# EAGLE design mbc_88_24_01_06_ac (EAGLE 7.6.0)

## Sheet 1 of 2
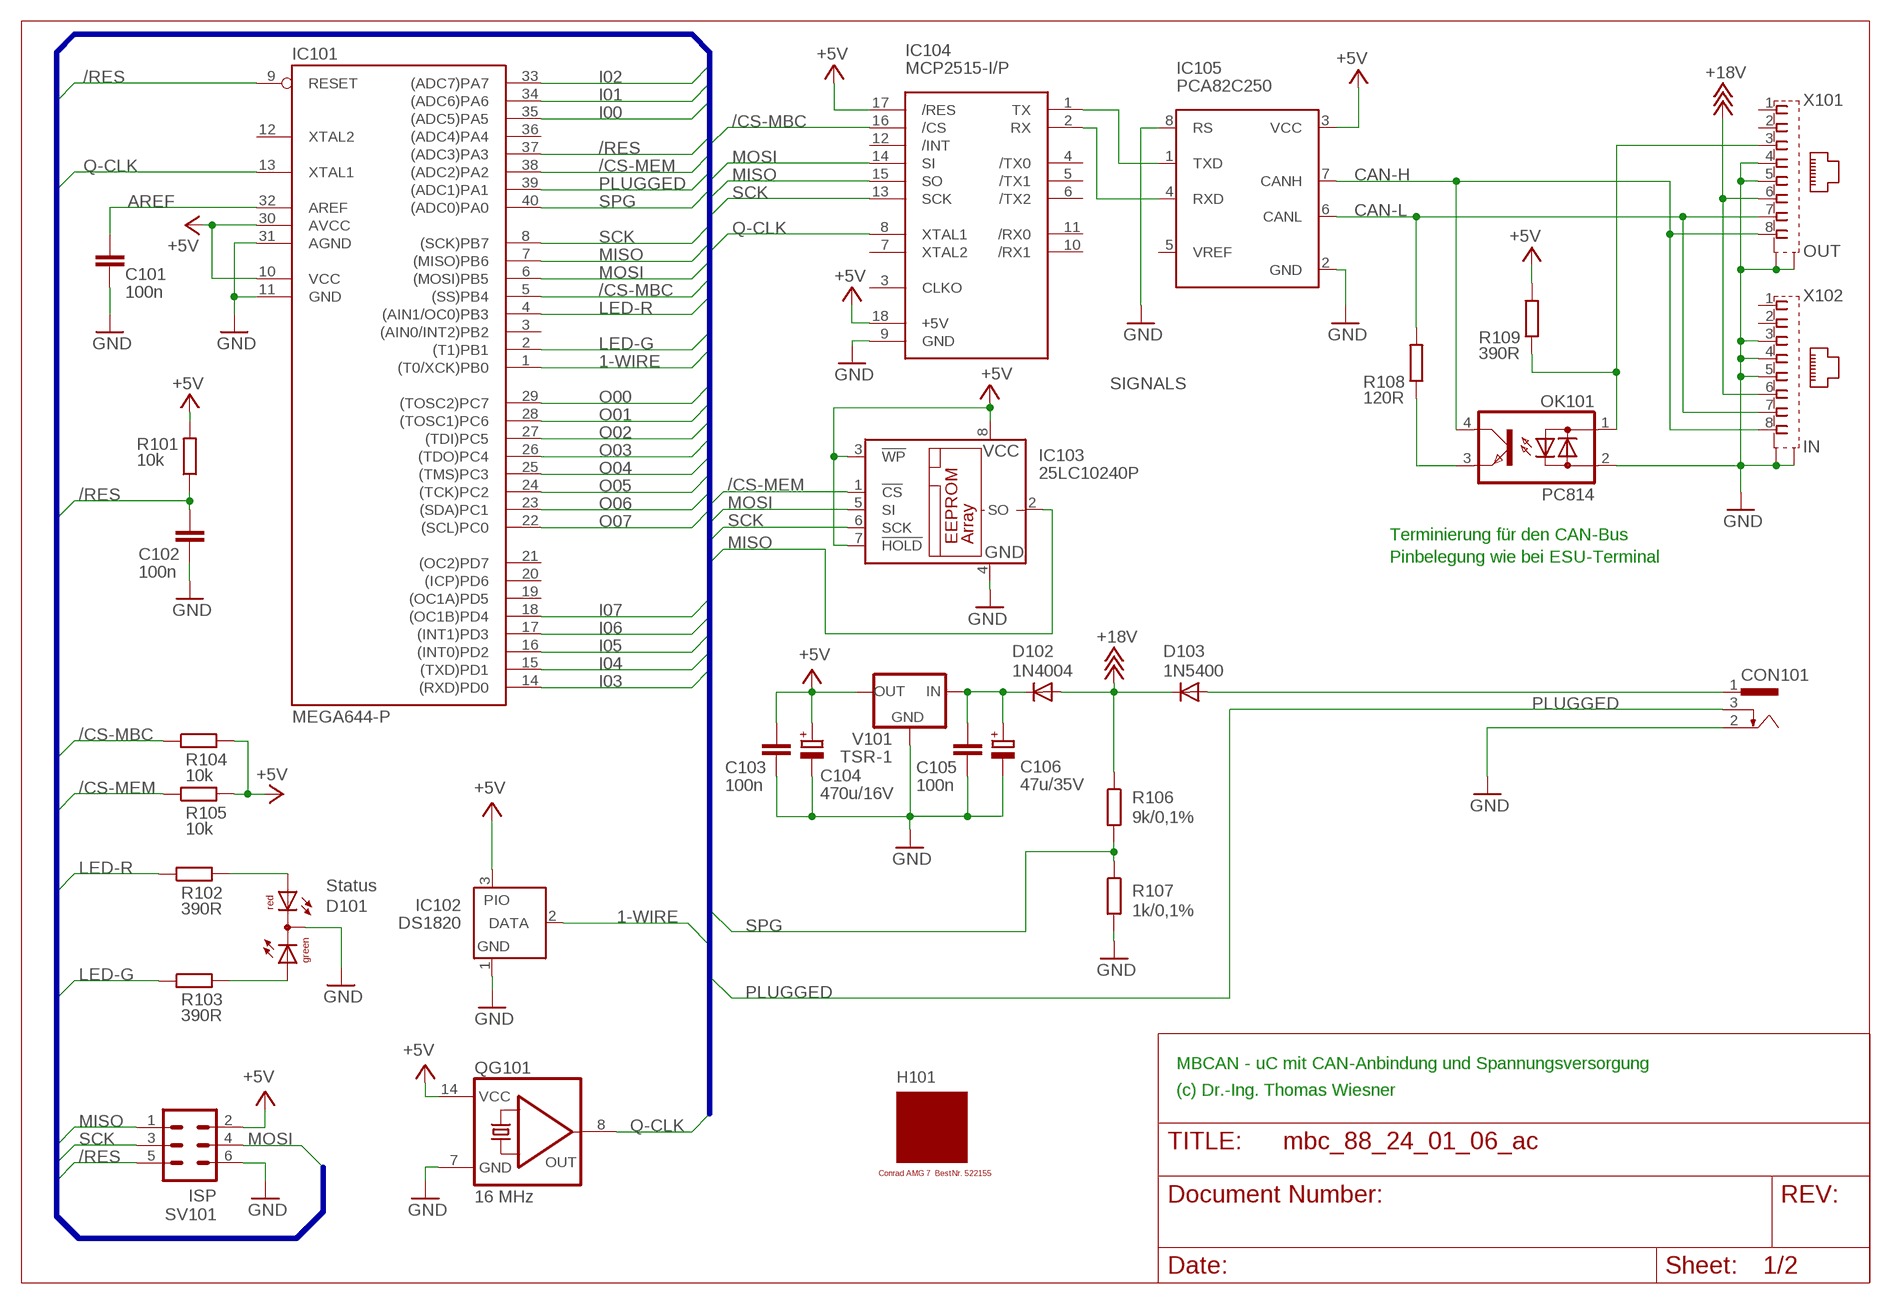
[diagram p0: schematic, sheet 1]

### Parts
C101  100n  C-EU025-025X050  [C025-025X050]
C102  100n  C-EU025-025X050  [C025-025X050]
C103  100n  C-EU025-025X050  [C025-025X050]
C104  470u/16V  CPOL-EUE3.5-8  [E3,5-8]
C105  100n  C-EU025-025X050  [C025-025X050]
C106  47u/35V  CPOL-EUE2.5-7  [E2,5-7]
CON101  POWER-JACK  [POWER-JACK]
D101  Status  DUOLED5MM  [DUOLED5MM]
D102  1N4004  [DO41-10]
D103  1N5400  [DO201-15]
H101  MODULGEHÄUSE-AMG-7  [MODULGEHÄUSE-1]
IC101  MEGA644-P  MEGA323-P  [DIL40]
IC102  DS1820  DS2405  [TO92-]
IC103  25LC10240P  25LC040P  [DIL8]
IC104  MCP2515-I/P  MCP2510-I/P  [DIL18]
IC105  PCA82C250  [DIL08]
OK101  PC814  [DIL04]
QG101  16 MHz  QG5860  [DIL14S]
R101  10k  R-EU_0207/10  [0207/10]
R102  390R  R-EU_0207/10  [0207/10]
R103  390R  R-EU_0207/10  [0207/10]
R104  10k  R-EU_0207/10  [0207/10]
R105  10k  R-EU_0207/10  [0207/10]
R106  9k/0,1%  R-EU_0207/10  [0207/10]
R107  1k/0,1%  R-EU_0207/10  [0207/10]
R108  120R  R-EU_0207/10  [0207/10]
R109  390R  R-EU_0207/10  [0207/10]
SV101  ISP  ML6  [ML6]
V101  TSR-1  [TRACO-TSR-1]
X101  OUT  0446200002  [0446200002]
X102  IN  0446200002  [0446200002]

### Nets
1-WIRE: IC101.1((T0/XCK)PB0) IC102.2(DATA)
+5V: C103.1 C104.+ IC101.10(VCC) IC101.30(AVCC) IC102.3(PIO) IC103.3(!WP) IC103.7(!HOLD) IC103.8(VCC) IC104.17(/RES) IC104.18(+5V) IC105.3(VCC) QG101.14(VCC) R101.2 R104.2 R105.2 R109.2 SV101.2 V101.OUT ; also sheet 2
+18V: D102.A D103.C R106.1 X101.6 X102.6
/CS-MBC: IC101.5((SS)PB4) IC104.16(/CS) R104.1
/CS-MEM: IC101.38((ADC2)PA2) IC103.1(!CS) R105.1
/RES: C102.1 IC101.9(RESET) IC101.37((ADC3)PA3) R101.1 SV101.5
AREF: C101.1 IC101.32(AREF)
CAN-H: IC105.7(CANH) OK101.4(C) X101.8 X102.8
CAN-L: IC105.6(CANL) R108.2 X101.7 X102.7
GND: C101.2 C102.2 C103.2 C104.- C105.2 C106.- CON101.2 D101.K(C) IC101.11(GND) IC101.31(AGND) IC102.1(GND) IC103.4(GND) IC104.9(GND) IC105.2(GND) IC105.8(RS) OK101.2(AC2) QG101.7(GND) R107.2 SV101.6 V101.GND X101.4 X101.5 X101.S@1(S1) X101.S@2(S2) X102.3 X102.4 X102.5 X102.S@1(S1) X102.S@2(S2) ; also sheet 2
I00: IC101.35((ADC5)PA5) ; also sheet 2
I01: IC101.34((ADC6)PA6) ; also sheet 2
I02: IC101.33((ADC7)PA7) ; also sheet 2
I03: IC101.14((RXD)PD0) ; also sheet 2
I04: IC101.15((TXD)PD1) ; also sheet 2
I05: IC101.16((INT0)PD2) ; also sheet 2
I06: IC101.17((INT1)PD3) ; also sheet 2
I07: IC101.18((OC1B)PD4) ; also sheet 2
LED-G: IC101.2((T1)PB1) R103.1
LED-R: IC101.4((AIN1/OC0)PB3) R102.1
MISO: IC101.7((MISO)PB6) IC103.2(SO) IC104.15(SO) SV101.1
MOSI: IC101.6((MOSI)PB5) IC103.5(SI) IC104.14(SI) SV101.4
N$1: IC104.1(TX) IC105.1(TXD)
N$2: IC104.2(RX) IC105.4(RXD)
N$3: OK101.1(AC1) R109.1 X101.3
N$5: OK101.3(E) R108.1
N$6: C105.1 C106.+ D102.C V101.IN
N$9: D101.AR R102.2
N$13: D101.AG R103.2
O00: IC101.29((TOSC2)PC7) ; also sheet 2
O01: IC101.28((TOSC1)PC6) ; also sheet 2
O02: IC101.27((TDI)PC5) ; also sheet 2
O03: IC101.26((TDO)PC4) ; also sheet 2
O04: IC101.25((TMS)PC3) ; also sheet 2
O05: IC101.24((TCK)PC2) ; also sheet 2
O06: IC101.23((SDA)PC1) ; also sheet 2
O07: IC101.22((SCL)PC0) ; also sheet 2
PLUGGED: CON101.3 IC101.39((ADC1)PA1)
Q-CLK: IC101.13(XTAL1) IC104.8(XTAL1) QG101.8(OUT)
SCK: IC101.8((SCK)PB7) IC103.6(SCK) IC104.13(SCK) SV101.3
SPG: IC101.40((ADC0)PA0) R106.2 R107.1
V-NETZTEIL1: CON101.1 D103.A
Unconnected: IC101.3((AIN0/INT2)PB2) IC101.12(XTAL2) IC101.19((OC1A)PD5) IC101.20((ICP)PD6) IC101.21((OC2)PD7) IC101.36((ADC4)PA4) IC104.3(CLKO) IC104.4(/TX0) IC104.5(/TX1) IC104.6(/TX2) IC104.7(XTAL2) IC104.10(/RX1) IC104.11(/RX0) IC104.12(/INT) IC105.5(VREF) X101.1 X101.2 X102.1 X102.2

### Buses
SIGNALS

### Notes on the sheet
- Terminierung für den CAN-Bus
- Pinbelegung wie bei ESU-Terminal
- MBCAN - uC mit CAN-Anbindung und Spannungsversorgung
- (c) Dr.-Ing. Thomas Wiesner

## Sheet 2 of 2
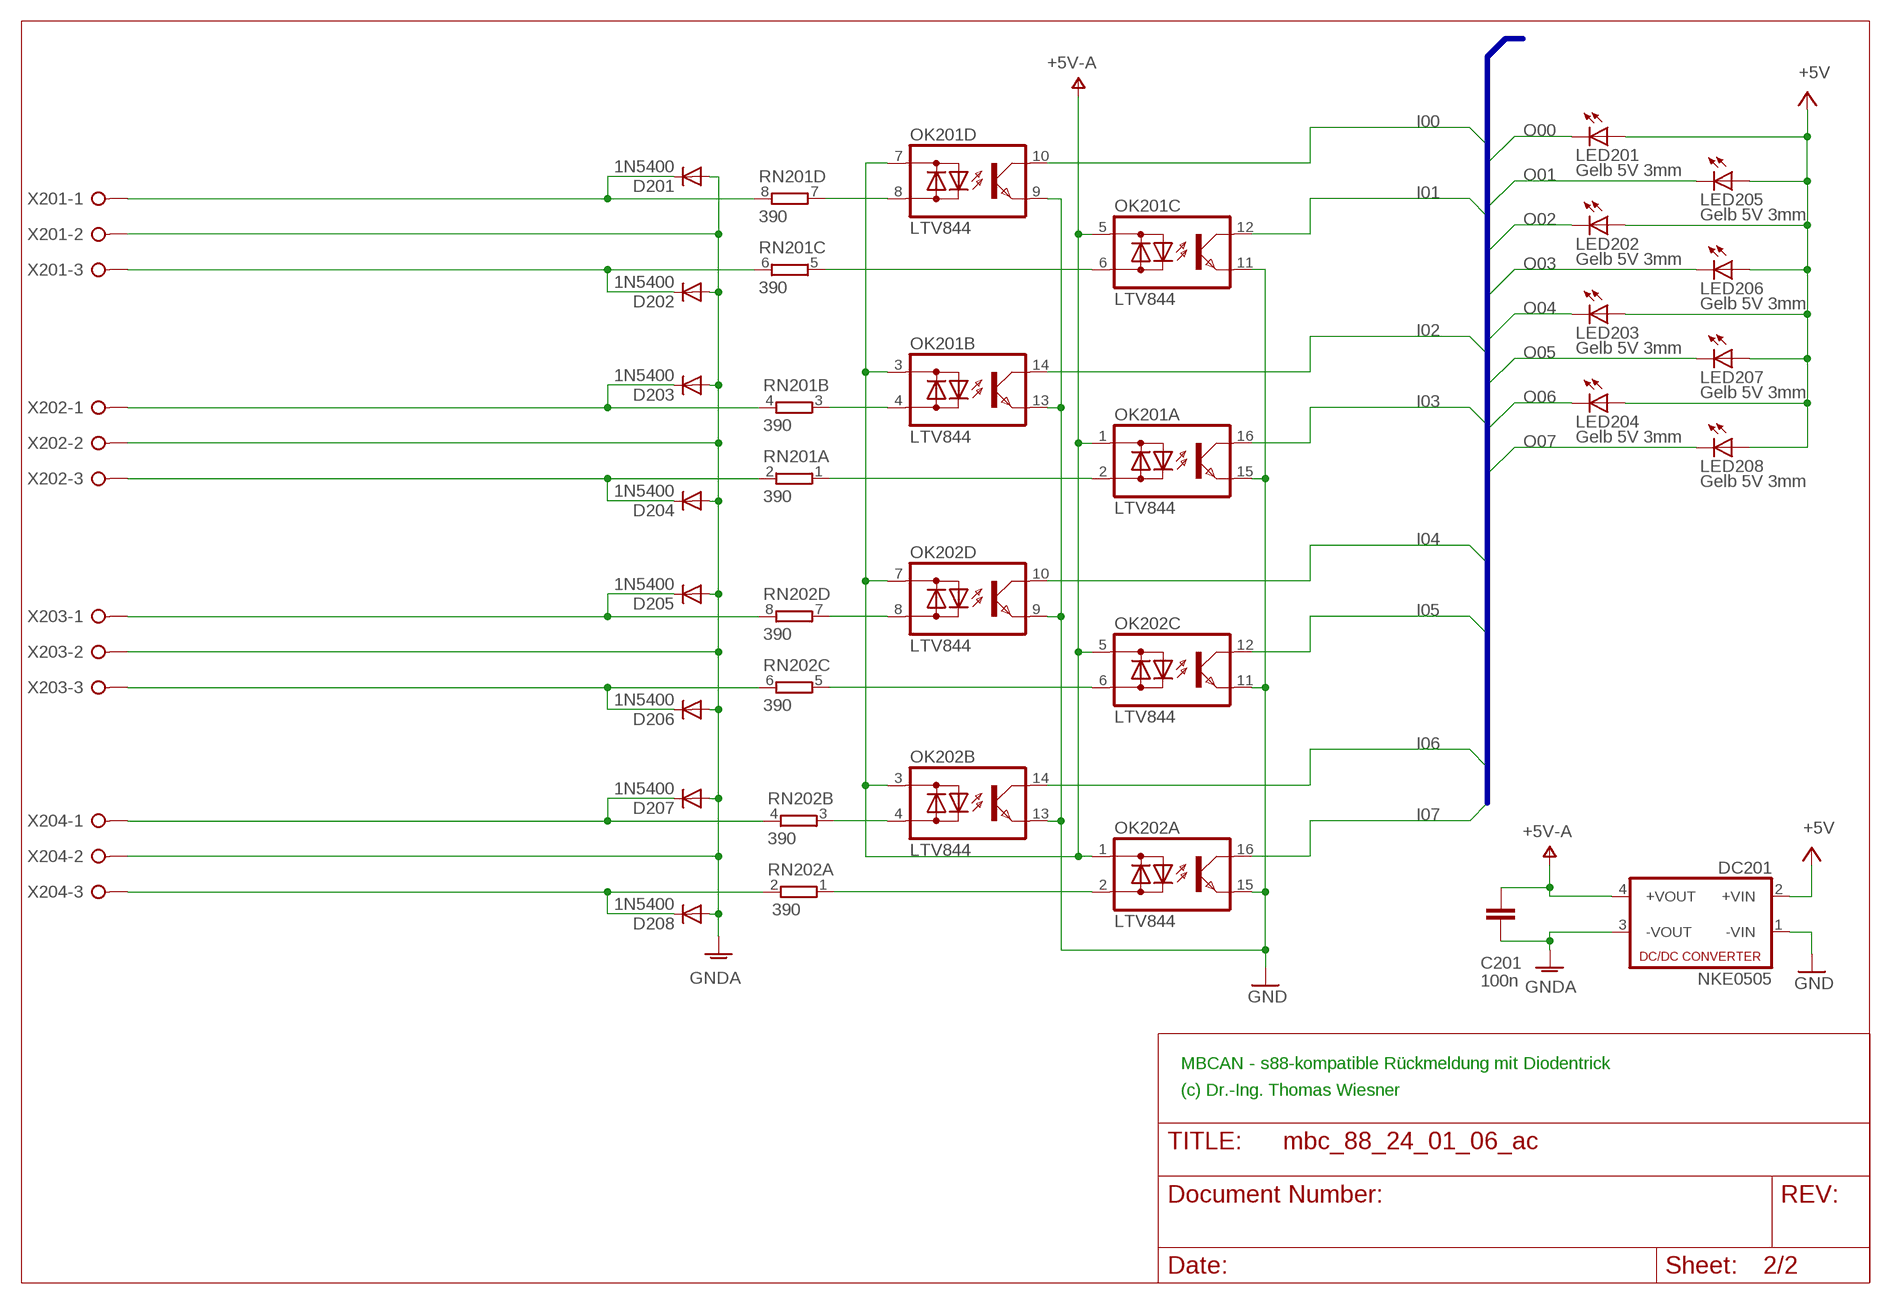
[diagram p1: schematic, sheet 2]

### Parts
C201  100n  C-EU025-025X050  [C025-025X050]
D201  1N5400  [DO201-15]
D202  1N5400  [DO201-15]
D203  1N5400  [DO201-15]
D204  1N5400  [DO201-15]
D205  1N5400  [DO201-15]
D206  1N5400  [DO201-15]
D207  1N5400  [DO201-15]
D208  1N5400  [DO201-15]
DC201  NKE0505  NME  [NME]
LED201  Gelb 5V 3mm  LED3MM  [LED3MM]
LED202  Gelb 5V 3mm  LED3MM  [LED3MM]
LED203  Gelb 5V 3mm  LED3MM  [LED3MM]
LED204  Gelb 5V 3mm  LED3MM  [LED3MM]
LED205  Gelb 5V 3mm  LED3MM  [LED3MM]
LED206  Gelb 5V 3mm  LED3MM  [LED3MM]
LED207  Gelb 5V 3mm  LED3MM  [LED3MM]
LED208  Gelb 5V 3mm  LED3MM  [LED3MM]
OK201  LTV844  TIL196  [DIL16]
OK202  LTV844  TIL196  [DIL16]
RN201  390  E4R  [SIL8]
RN202  390  E4R  [SIL8]
X201  W237-03P  [W237-133]
X202  W237-03P  [W237-133]
X203  W237-03P  [W237-133]
X204  W237-03P  [W237-133]

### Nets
+5V: DC201.2(+VIN) LED201.A LED202.A LED203.A LED204.A LED205.A LED206.A LED207.A LED208.A ; also sheet 1
GND: DC201.1(-VIN) OK201.9(D:E) OK201.11(C:E) OK201.13(B:E) OK201.15(A:E) OK202.9(D:E) OK202.11(C:E) OK202.13(B:E) OK202.15(A:E) ; also sheet 1
GNDA: C201.2 D201.A D202.A D203.A D204.A D205.A D206.A D207.A D208.A DC201.3(-VOUT) X201.2 X202.2 X203.2 X204.2
I00: OK201.10(D:C) ; also sheet 1
I01: OK201.12(C:C) ; also sheet 1
I02: OK201.14(B:C) ; also sheet 1
I03: OK201.16(A:C) ; also sheet 1
I04: OK202.10(D:C) ; also sheet 1
I05: OK202.12(C:C) ; also sheet 1
I06: OK202.14(B:C) ; also sheet 1
I07: OK202.16(A:C) ; also sheet 1
N$24: D207.C RN202.4 X204.1
N$25: D208.C RN202.2 X204.3
N$26: D205.C RN202.8 X203.1
N$27: D206.C RN202.6 X203.3
N$28: D203.C RN201.4 X202.1
N$29: D204.C RN201.2 X202.3
N$30: D201.C RN201.8 X201.1
N$42: OK202.2(A:AC2) RN202.1
N$43: OK202.4(B:AC2) RN202.3
N$44: OK202.6(C:AC2) RN202.5
N$45: OK202.8(D:AC2) RN202.7
N$46: OK201.2(A:AC2) RN201.1
N$47: D202.C RN201.6 X201.3
N$48: OK201.4(B:AC2) RN201.3
N$64: OK201.6(C:AC2) RN201.5
N$65: OK201.8(D:AC2) RN201.7
O00: LED201.K(C) ; also sheet 1
O01: LED205.K(C) ; also sheet 1
O02: LED202.K(C) ; also sheet 1
O03: LED206.K(C) ; also sheet 1
O04: LED203.K(C) ; also sheet 1
O05: LED207.K(C) ; also sheet 1
O06: LED204.K(C) ; also sheet 1
O07: LED208.K(C) ; also sheet 1
V+: C201.1 DC201.4(+VOUT) OK201.1(A:AC1) OK201.3(B:AC1) OK201.5(C:AC1) OK201.7(D:AC1) OK202.1(A:AC1) OK202.3(B:AC1) OK202.5(C:AC1) OK202.7(D:AC1) ; supply symbol labelled +5V-A

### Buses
B$1

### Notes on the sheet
- MBCAN - s88-kompatible Rückmeldung mit Diodentrick
- (c) Dr.-Ing. Thomas Wiesner

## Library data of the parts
C101-C103 C105 C201 = rcl:C-EU: CAPACITOR, European symbol
C104 C106 = rcl:CPOL-EU: POLARIZED CAPACITOR, European symbol
CON101 = mbc:POWER-JACK: Power-Stecker für 2,5 mm Hohlbuchse
D101 = led:DUOLED5MM: DUO LED 2 colors, 5 mm, round
D102 = diode:1N4004: DIODE
D103 D201-D208 = diode:1N5400: DIODE
DC201 = dc-dc-converter:NME: DC-DC CONVERTER; MF: C & D TECHNOLOGIES, INC; MPN: NME1205D; OC_FARNELL: 1021466; OC_NEWARK: 98B8198
H101 = mbc:MODULGEHÄUSE-AMG-7: Gehäuse
IC101 = atmel:MEGA323-P: MICROCONTROLLER 32 Kbytes FLASH 2 Kbytes SRAM 1 Kbytes EEPROM USART 8-channel 10 bit ADC Source: avr.lbr; OC_FARNELL: unknown; OC_NEWARK: unknown
IC102 = maxim:DS2405: Addressable Switch DALLAS Semiconductor; MF: DALLAS SEMICONDUCTOR; MPN: DS2405; OC_FARNELL: 1188025; OC_NEWARK: 06F4645
IC103 = microchip:25*: Serial EEPROM 4K/ 8K , SPI bus; MF: MICROCHIP; MPN: 25LC040/P; OC_FARNELL: 9758100; OC_NEWARK: 96K4091
IC104 = mbc:MCP2510: BASIC-CAN 2.0a Controller Stand-alone CAN controller von Microchip
IC105 = micro-philips:PCA82C250: CAN CONTROLLER INTERFACE; OC_FARNELL: 3692358; OC_NEWARK: unknown
LED201-LED208 = led:LED: LED
OK101 = optocoupler:PC814: SHARP OPTO COUPLER; OC_FARNELL: 9707662; OC_NEWARK: unknown
OK201 OK202 = optocoupler:TIL196: TEXAS INSTRUMENTS OPTO COUPLER; MPN: TIL 196; OC_FARNELL: 1683367; OC_NEWARK: 05R6476
QG101 = crystal:QG5860: CRYSTAL RESONATOR; OC_FARNELL: unknown; OC_NEWARK: unknown
R101-R109 = resistor:R-EU_: RESISTOR, European symbol
RN201 RN202 = resistor-sil:E4R: SIL RESISTOR; OC_FARNELL: unknown; OC_NEWARK: unknown
SV101 = con-ml:ML6: HARTING; OC_FARNELL: unknown; OC_NEWARK: unknown
V101 = mbc:TSR-1: Spannungsregler Hersteller: TRACO Typ: TSR-1 5V: TSR 1-2450 Spg: 5V Strom: 1A Reichelt TSR 1-2450
X101 X102 = mbc:0446200002: RJ-45 INVERTED MODULAR JACK ASSEMBLY WITH RJ-11 KEEPOUT FEATURE Source: Data sheet MOLEX 0446200002 BUCHSE, RJ45, GESCHIRMT Source: Farnell; MF: MOLEX; MPN: 0446200002; OC_FARNELL: 9251910
X201-X204 = con-wago-508:W237-03P: WAGO SREW CLAMP; OC_FARNELL: unknown; OC_NEWARK: unknown

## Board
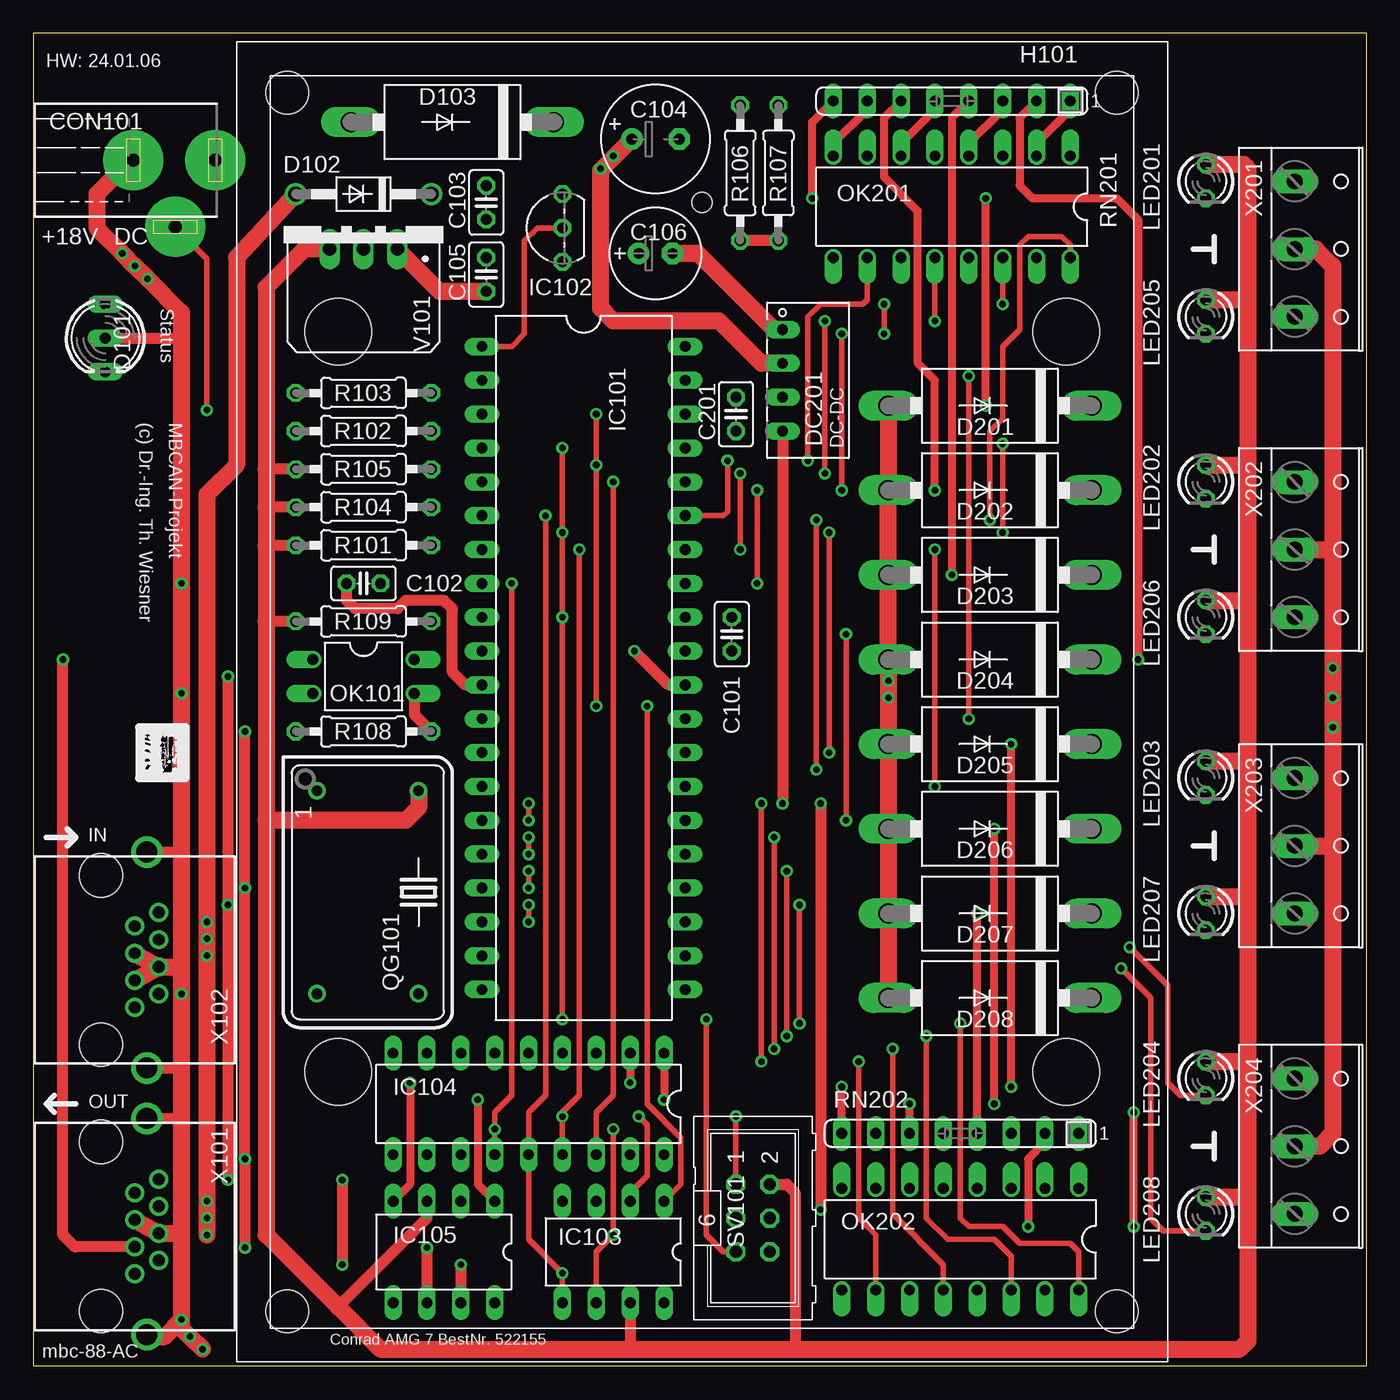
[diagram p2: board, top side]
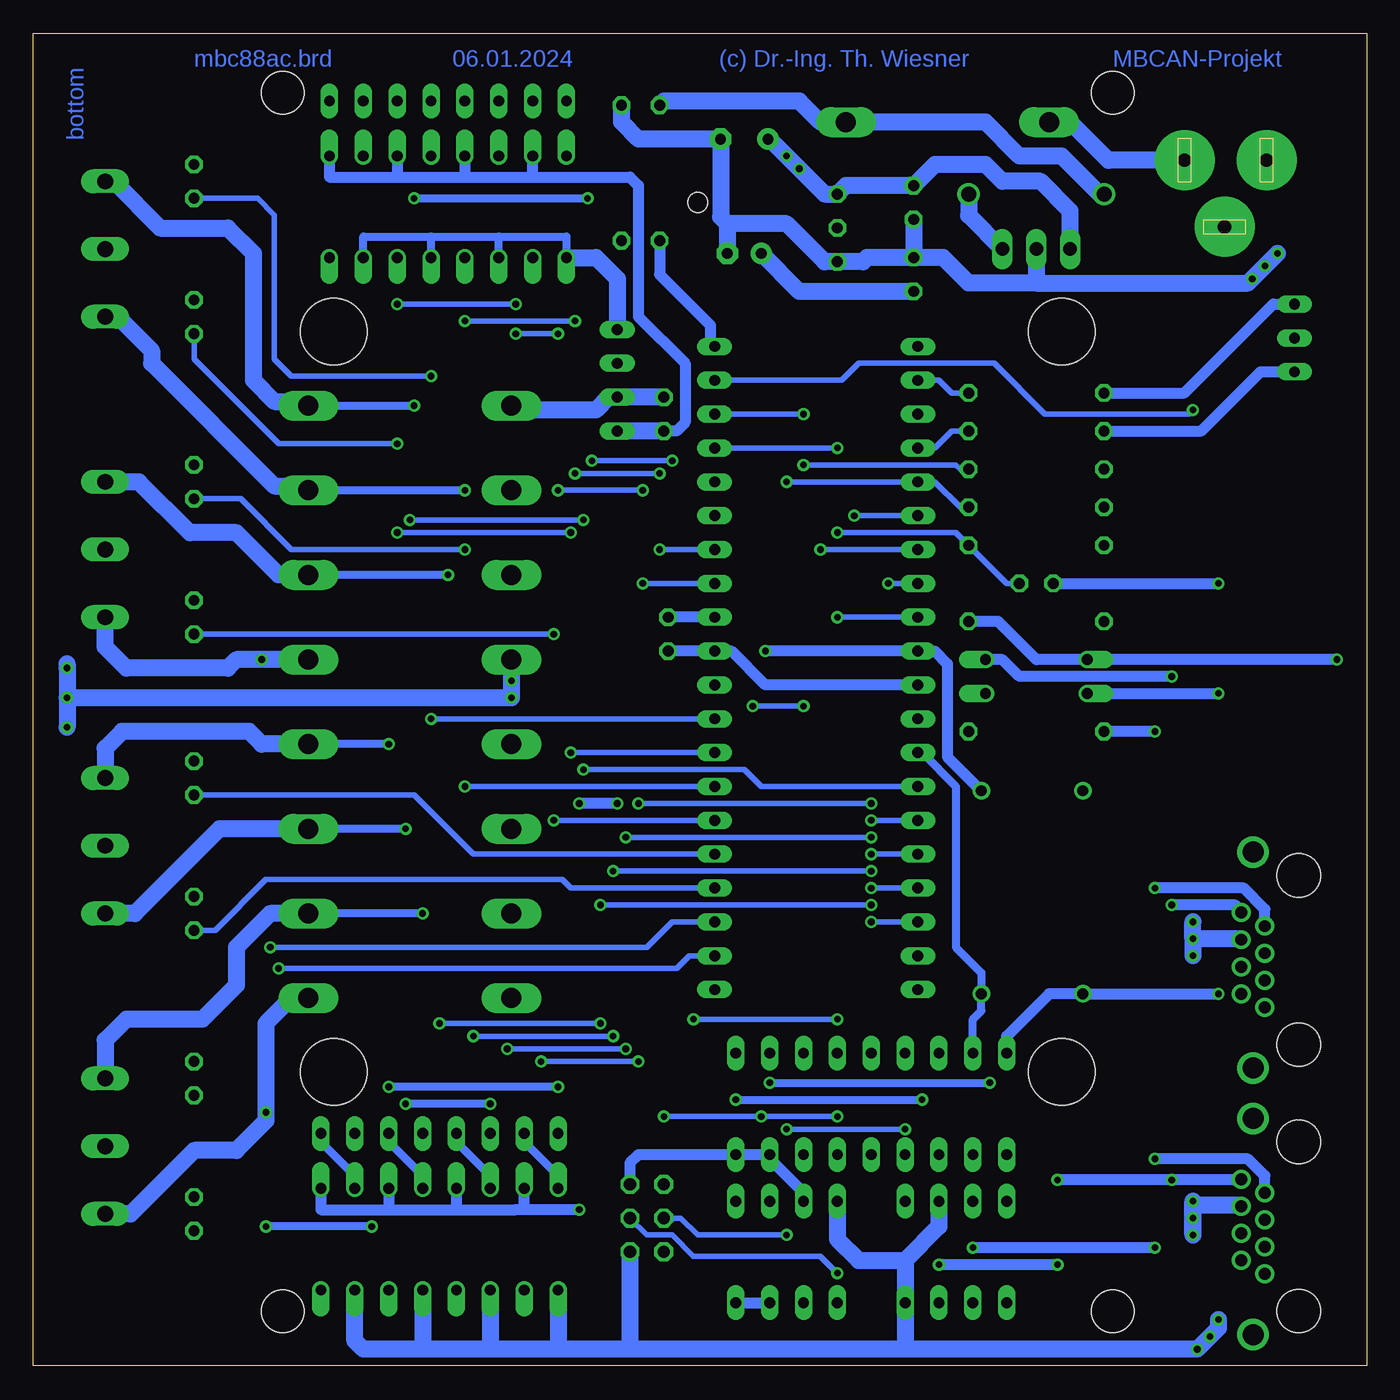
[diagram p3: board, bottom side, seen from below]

Size 100 x 99.99 mm. Coordinates in mm from the lower left corner, seen from the top.
Outline: 0,99.99 0,0 100,0 100,99.99 0,99.99
Copper layers (1*16): Top 0.035mm / dielectric 1.5mm / Bottom 0.035mm
Design rules "default *": minimum track width 10mil, minimum drill 0.5mm, track to track 8mil, track to pad 8mil, pad to pad 8mil, via to via 8mil, smd to smd 8mil, copper to edge 40mil, drill to drill 8mil, minimum pad ring 10mil, minimum via ring 8mil, stop-mask expansion 4mil, vias tented up to drill 0mil, thermal gap 10mil

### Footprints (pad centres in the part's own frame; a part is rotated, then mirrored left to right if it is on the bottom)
C025-025X050 = drill 0.813 octagon: 1 -1.27,0; 2 1.27,0
E3,5-8 = drill 0.813 pad 1.6: + -1.778,0 | drill 0.813 pad 1.6 octagon: - 1.778,0
E2,5-7 = drill 0.813 pad 1.6: + -1.27,0 | drill 0.813 pad 1.6 octagon: - 1.27,0
POWER-JACK = drill 1 pad 4.5: 1 0,6.03; 2 0,-0.12; 3 5,3.03
DUOLED5MM = drill 0.813 long: AG -2.54,0; AR 2.54,0; K 0,0
DO41-10 = drill 1.118: A 5.08,0; C -5.08,0
DO201-15 = drill 1.499 long: A 7.62,0; C -7.62,0
NME = drill 0.813 long: 1 0,3.81; 2 0,1.27; 3 0,-1.27; 4 0,-3.81
MODULGEHÄUSE-1 = hole 3.2: -45.72,-31.115; -45.72,31.115; 45.72,31.115; 45.72,-31.115 | hole 5: -27.781,-27.305; 27.781,-27.305; -27.781,27.305; 27.781,27.305 | hole 1.5: -37.465,0
DIL40 = drill 0.813 long: 1 -24.13,-7.62; 2 -21.59,-7.62; 3 -19.05,-7.62; 4 -16.51,-7.62; 5 -13.97,-7.62; 6 -11.43,-7.62; 7 -8.89,-7.62; 8 -6.35,-7.62; 9 -3.81,-7.62; 10 -1.27,-7.62; 11 1.27,-7.62; 12 3.81,-7.62; 13 6.35,-7.62; 14 8.89,-7.62; 15 11.43,-7.62; 16 13.97,-7.62; 17 16.51,-7.62; 18 19.05,-7.62; 19 21.59,-7.62; 20 24.13,-7.62; 21 24.13,7.62; 22 21.59,7.62; 23 19.05,7.62; 24 16.51,7.62; 25 13.97,7.62; 26 11.43,7.62; 27 8.89,7.62; 28 6.35,7.62; 29 3.81,7.62; 30 1.27,7.62; 31 -1.27,7.62; 32 -3.81,7.62; 33 -6.35,7.62; 34 -8.89,7.62; 35 -11.43,7.62; 36 -13.97,7.62; 37 -16.51,7.62; 38 -19.05,7.62; 39 -21.59,7.62; 40 -24.13,7.62
TO92- = drill 0.813 octagon: 1 -2.54,0; 2 0,0; 3 2.54,0
DIL8 = drill 0.813 long: 1 -3.81,-3.81; 2 -1.27,-3.81; 3 1.27,-3.81; 4 3.81,-3.81; 5 3.81,3.81; 6 1.27,3.81; 7 -1.27,3.81; 8 -3.81,3.81
DIL18 = drill 0.813 long: 1 -10.16,-3.81; 2 -7.62,-3.81; 3 -5.08,-3.81; 4 -2.54,-3.81 | drill 0.8 long: 5 0,-3.81; 6 2.54,-3.81; 7 5.08,-3.81; 8 7.62,-3.81; 9 10.16,-3.81; 10 10.16,3.81; 11 7.62,3.81; 12 5.08,3.81; 13 2.54,3.81; 14 0,3.81; 15 -2.54,3.81; 16 -5.08,3.81; 17 -7.62,3.81; 18 -10.16,3.81
DIL08 = drill 0.813 long: 1 -3.81,-3.81; 2 -1.27,-3.81; 3 1.27,-3.81; 4 3.81,-3.81; 5 3.81,3.81; 6 1.27,3.81; 7 -1.27,3.81; 8 -3.81,3.81
LED3MM = drill 0.813 octagon: A -1.27,0; K 1.27,0
DIL04 = drill 0.813 offset: 1 -1.27,-3.81; 2 1.27,-3.81; 3 1.27,3.81; 4 -1.27,3.81
DIL16 = drill 0.813 offset: 1 -8.89,-3.81; 2 -6.35,-3.81; 3 -3.81,-3.81; 4 -1.27,-3.81; 5 1.27,-3.81; 6 3.81,-3.81; 7 6.35,-3.81; 8 8.89,-3.81; 9 8.89,3.81; 10 6.35,3.81; 11 3.81,3.81; 12 1.27,3.81; 13 -1.27,3.81; 14 -3.81,3.81; 15 -6.35,3.81; 16 -8.89,3.81
DIL14S = drill 0.813: 1 -7.62,-3.81; 7 7.62,-3.81; 8 7.62,3.81; 14 -7.62,3.81
0207/10 = drill 0.813 octagon: 1 -5.08,0; 2 5.08,0
SIL8 = drill 0.813 long: 1 -8.89,0; 2 -6.35,0; 3 -3.81,0; 4 -1.27,0; 5 1.27,0; 6 3.81,0; 7 6.35,0; 8 8.89,0
ML6 = drill 0.914 octagon: 1 -2.54,-1.27; 2 -2.54,1.27; 3 0,-1.27; 4 0,1.27; 5 2.54,-1.27; 6 2.54,1.27
TRACO-TSR-1 = drill 1.016 long: GND 0,2.54; IN -2.54,2.54; OUT 2.54,2.54
0446200002 = drill 0.889 pad 1.422: 1 3.556,2.54; 2 2.54,4.318; 3 1.524,2.54; 4 0.508,4.318; 5 -0.508,2.54; 6 -1.524,4.318; 7 -2.54,2.54; 8 -3.556,4.318 | drill 1.575 pad 2.286: S@1 -8.103,3.429; S@2 8.103,3.429 | hole 3.251: 6.35,0; -6.35,0
W237-133 = drill 1.194 long: 1 -5.08,-0.635; 2 0,-0.635; 3 5.08,-0.635

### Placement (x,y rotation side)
C101  52.39,54.91 270 top
C102  24.77,58.72 180 top
C103  33.97,87.29 270 top
C104  46.67,92.06 0 top
C105  33.97,81.9 90 top
C106  46.67,83.48 0 top
C201  52.7,71.42 90 top
CON101  7.62,90.47 270 top
D101  5.4,77.13 270 top
D102  24.77,87.93 180 top
D103  31.43,93.33 180 top
D201  71.75,72.05 180 top
D202  71.75,65.7 180 top
D203  71.75,59.35 180 top
D204  71.75,53 180 top
D205  71.75,46.65 180 top
D206  71.75,40.3 180 top
D207  71.75,33.95 180 top
D208  71.75,27.6 180 top
DC201  56.2,73.96 0 top
H101  50.16,49.83 270 top
IC101  41.27,52.37 270 top
IC102  39.69,85.39 90 top
IC103  43.5,8.55 180 top
IC104  37.15,19.66 180 top
IC105  30.8,8.55 180 top
LED201  87.95,88.88 270 top
LED202  87.95,66.34 270 top
LED203  87.95,44.11 270 top
LED204  87.95,21.57 270 top
LED205  87.95,78.72 270 top
LED206  87.95,56.18 270 top
LED207  87.95,33.95 270 top
LED208  87.95,11.41 270 top
OK101  24.77,51.73 270 top
OK201  68.9,86.98 180 top
OK202  69.53,9.51 180 top
QG101  25.08,35.54 270 top
R101  24.77,61.57 180 top
R102  24.77,70.15 180 top
R103  24.77,73.01 180 top
R104  24.77,64.43 180 top
R105  24.77,67.29 180 top
R106  53.02,89.52 270 top
R107  55.88,89.52 90 top
R108  24.77,47.6 180 top
R109  24.77,55.86 180 top
RN201  68.9,94.91 180 top
RN202  69.53,17.44 180 top
SV101  53.98,11.09 270 top
V101  24.77,86.34 180 top
X101  5.08,10.46 270 top
X102  5.08,30.46 270 top
X201  95.25,83.8 270 top
X202  95.25,61.26 270 top
X203  95.25,39.03 270 top
X204  95.25,16.49 270 top

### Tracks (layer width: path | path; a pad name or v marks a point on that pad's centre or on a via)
1-WIRE
  Top 0.406: IC102.2 37.78,85.39 36.83,84.44 36.83,77.45 35.88,76.5 IC101.1
+5V  (via drill 0.5)
  Top 0.813: R104.2 17.46,64.43 | R101.2 17.46,61.57 | R105.2 17.46,67.29 | R109.2 17.46,55.86 | v45.09,53.64 47.62,51.1 IC101.30 | IC103.7 44.77,1.57 44.45,1.25 | SV101.2 56.52,13.63 57.15,13 57.15,1.25 | IC105.3 29.53,11.09 22.86,4.43
  Top 1.27: V101.OUT 20.32,83.8 17.46,80.94 17.46,67.29 17.46,64.43 17.46,61.57 17.46,55.86 17.46,40.94 | 17.46,40.94 17.46,9.82 22.86,4.43 26.04,1.25 44.45,1.25 57.15,1.25 90.49,1.25 91.12,1.89 91.12,12.68 | 91.12,12.68 91.12,23.16 | 91.12,23.16 91.12,35.54 | 91.12,35.54 91.12,45.38 | 91.12,45.38 91.12,57.45 | 91.12,57.45 91.12,67.61 | 91.12,67.61 91.12,80.31 | 91.12,80.31 91.12,89.83 90.81,90.15 LED201.A | LED205.A 90.81,79.99 91.12,80.31 | LED202.A 91.12,67.61 | LED206.A 91.12,57.45 | LED203.A 91.12,45.38 | LED207.A 90.81,35.22 91.12,35.54 | LED204.A 90.81,22.84 91.12,23.16 | LED208.A 91.12,12.68 | QG101.14 28.89,41.89 27.94,40.94 17.46,40.94 | DC201.2 54.61,75.23 51.44,78.4 43.5,78.4 42.55,79.36 42.55,89.7 C104.+
  Bottom 0.813: v45.09,53.64 IC101.10 32.38,53.64 31.43,52.68 31.43,45.7 QG101.14 | IC103.3 42.23,13 44.77,15.54 IC104.17 IC104.18 54.61,15.86 55.24,15.22 SV101.2 | IC103.8 IC103.7
  Bottom 1.27: C104.+ 44.77,92.06 v43.5,90.79 v42.55,89.83 40.64,87.93 IC102.3 39.05,88.56 C103.1 32.38,90.15 28.57,90.15 27.3,88.88 24.45,88.88 22.23,86.66 V101.OUT
+18V  (via drill 0.5)
  Top 1.27: D102.A 15.24,83.17 15.24,67.61 13.02,65.39 v13.02,33.32 v13.02,32.05 v13.02,30.78 v13.02,12.36 v13.02,11.09 v13.02,9.82
  Bottom 1.27: X101.6 9.4,12.04 13.02,12.04 v13.02,9.82 v13.02,11.09 v13.02,12.36 | X102.6 9.4,32.05 v13.02,32.05 | v13.02,32.05 v13.02,33.32 | v13.02,32.05 v13.02,30.78 | D102.A 20,87.93 22.86,90.79 26.04,90.79 28.57,93.33 D103.C 40.96,93.33 42.55,94.91 52.7,94.91 R106.1
/CS-MBC  (via drill 0.5)
  Top 0.406: IC104.16 42.23,19.03 43.5,20.3 v43.5,66.34
  Bottom 0.406: v43.5,66.34 IC101.5 32.38,66.34 30.48,64.43 R104.1
/CS-MEM  (via drill 0.5)
  Top 0.406: v42.23,71.42 v42.23,67.61 v42.23,49.51 | IC103.1 48.58,13.63 48.58,17.12 46.04,19.66 v46.04,49.51
  Bottom 0.406: R105.1 30.48,67.29 30.8,67.61 v42.23,67.61 | v42.23,71.42 IC101.38 | v46.04,49.51 v42.23,49.51
/RES  (via drill 0.5)
  Top 0.406: v39.69,26.02 v39.69,56.18 v39.69,62.53 v39.69,68.88 | v50.48,26.02 50.48,9.82 51.75,8.55 SV101.5
  Bottom 0.406: C102.1 26.99,58.72 R101.1 30.8,62.53 v39.69,62.53 | v39.69,26.02 v50.48,26.02 | v39.69,68.88 IC101.37 | IC101.9 v39.69,56.18
AREF
  Bottom 0.813: IC101.32 C101.1
CAN-H  (via drill 0.5)
  Top 0.813: v14.61,13.95 v14.61,34.59 v14.61,51.73 | v23.18,13.95 v23.18,7.6 | v32.07,7.6 IC105.7
  Bottom 0.813: X101.8 9.4,13.95 v14.61,13.95 v23.18,13.95 | v14.61,51.73 26.04,51.73 27.3,53 OK101.4 | X102.8 9.4,34.14 9.84,34.59 v14.61,34.59 | v23.18,7.6 v32.07,7.6
CAN-L  (via drill 0.5)
  Top 0.813: v15.88,47.6 v15.88,35.86 v15.88,15.54 v15.88,8.87 | v29.53,8.87 IC105.6
  Bottom 0.813: X101.7 7.62,14.27 8.89,15.54 v15.88,15.54 | v15.88,47.6 R108.2 | X102.7 7.62,34.27 9.21,35.86 v15.88,35.86 | v15.88,8.87 v29.53,8.87
GND  (via drill 0.5)
  Top 0.813: X101.S@1 10.64,18.56 11.11,19.03 | X102.S@1 10.64,38.56 11.11,39.03 | D101.K 10.79,77.13 11.11,76.81 | IC101.11 32.38,51.1 31.43,52.05 31.43,56.81 30.8,57.45 27.94,57.45 27.3,56.81 24.13,56.81 23.5,57.45 C102.2 | X102.S@2 10.95,22.36 11.11,22.52
  Top 1.27: CON101.2 7.3,90.47 4.76,87.93 4.76,85.39 v6.67,83.48 v7.62,82.53 v8.57,81.58 11.11,79.04 11.11,76.81 v11.11,58.72 v11.11,50.46 11.11,39.03 11.11,30.14 | 11.11,30.14 v11.11,27.92 11.11,22.52 11.11,19.03 11.11,9.82 | 11.11,9.82 v11.11,3.47 | v11.11,3.47 11.11,2.84 v11.75,2.2 v12.7,1.25 | v11.11,3.47 9.84,2.2 8.66,2.2 X101.S@2 | X102.4 10.92,29.95 arc90 11.11,30.14 | 11.11,9.82 arc90 10.99,9.95 X101.4 X101.5 | X102.5 X102.4 | X102.3 X102.4 | C106.- 49.85,83.48 55.56,77.77 DC201.1
  Bottom 0.61: OK201.15 75.25,84.75 70.17,84.75 | 70.17,84.75 65.09,84.75 | 65.09,84.75 60.01,84.75 OK201.9 | OK201.11 65.09,84.75 | OK201.13 70.17,84.75
  Bottom 0.813: v11.11,27.92 QG101.7 23.81,27.92 26.99,24.75 IC104.9 | OK101.2 v11.11,50.46 | IC101.11 45.09,51.1 47.62,53.64 IC101.31 C101.2 | C102.2 v11.11,58.72
  Bottom 1.27: 34.61,1.25 v12.7,1.25 11.11,2.84 v11.11,3.47 | 34.61,1.25 55.24,1.25 | 55.24,1.25 60.96,1.25 | 60.96,1.25 65.72,1.25 | 65.72,1.25 70.8,1.25 | 70.8,1.25 75.25,1.25 75.88,1.89 OK202.15 | 24.77,81.26 8.89,81.26 v8.57,81.58 v7.62,82.53 v6.67,83.48 | V101.GND 24.77,81.26 | 24.77,81.26 29.84,81.26 31.75,83.17 C105.2 | C105.2 37.47,83.17 37.78,82.85 IC102.1 40.64,82.85 43.5,85.7 47.94,85.7 | C103.2 C105.2 | 47.94,85.7 C106.- | 47.94,85.7 48.45,86.21 C104.- 54.61,92.06 55.88,93.33 R107.2 | OK201.9 57.78,83.17 56.2,81.58 DC201.1 | OK202.13 70.8,1.25 | OK202.11 65.72,1.25 | OK202.9 60.64,1.57 60.96,1.25 | SV101.6 55.24,1.25 | 34.61,1.25 IC105.8 34.61,7.92 | IC105.2 32.07,10.46 34.61,7.92 | IC103.4 39.69,9.51 38.1,7.92 34.61,7.92
GNDA  (via drill 0.5)
  Top 1.27: D201.A D202.A D203.A D204.A v64.14,51.41 v64.14,50.14 D205.A D206.A D207.A D208.A | X201.2 96.2,83.8 97.47,82.53 97.47,61.26 | 97.47,61.26 v97.47,52.37 v97.47,50.14 v97.47,47.92 97.47,39.35 | 97.47,39.35 97.47,17.44 96.52,16.49 X204.2 | X203.2 97.16,39.03 97.47,39.35 | X202.2 97.47,61.26
  Bottom 1.27: 97.47,52.68 v97.47,52.37 v97.47,50.14 | v97.47,50.14 v97.47,47.92 | v97.47,50.14 v64.14,50.14 v64.14,51.41 D204.A | C201.2 DC201.3 56.83,72.69 57.78,71.73 63.82,71.73 D201.A
I00  (via drill 0.5)
  Top 0.406: OK201.10 62.55,79.99 62.23,79.67 59.05,79.67 58.1,78.72 v58.1,67.92 | v52.07,67.92 52.07,64.12 51.75,63.8 IC101.35
  Bottom 0.406: v58.1,67.92 v52.07,67.92
I01  (via drill 0.5)
  Top 0.406: OK201.12 v67.63,78.4 | v59.37,78.4 v59.37,66.97 | v53.02,66.97 v53.02,61.26
  Bottom 0.406: v67.63,78.4 v59.37,78.4 | v59.37,66.97 v53.02,66.97 | v53.02,61.26 IC101.34
I02  (via drill 0.5)
  Top 0.406: OK201.14 v72.71,79.67 | v63.82,79.67 v63.82,77.45 | v60.64,77.45 v60.64,65.7 | v54.29,65.7 v54.29,58.72
  Bottom 0.406: v72.71,79.67 v63.82,79.67 | v63.82,77.45 v60.64,77.45 | v60.64,65.7 v54.29,65.7 | v54.29,58.72 IC101.33
I03  (via drill 0.5)
  Top 0.406: v58.74,44.75 v58.74,63.48 | v71.75,63.48 71.75,70.15 72.71,71.1 72.71,76.5 73.98,77.77 73.98,84.12 74.61,84.75 77.15,84.75 77.79,84.12 OK201.16
  Bottom 0.406: IC101.14 45.4,43.48 46.67,44.75 v58.74,44.75 | v58.74,63.48 v71.75,63.48
I04  (via drill 0.5)
  Top 0.406: OK202.10 63.18,9.82 61.91,11.09 v61.91,22.84 | v54.61,22.84 v54.61,42.21 | v37.15,42.21 v37.15,40.94
  Bottom 0.406: v61.91,22.84 v54.61,22.84 | v54.61,42.21 v37.15,42.21 | v37.15,40.94 IC101.15
I05  (via drill 0.5)
  Top 0.406: OK202.12 68.26,7.6 64.45,11.41 v64.45,23.79 | v55.56,23.79 v55.56,39.67 | v37.15,39.67 v37.15,38.4
  Bottom 0.406: v64.45,23.79 v55.56,23.79 | v55.56,39.67 v37.15,39.67 | v37.15,38.4 IC101.16
I06  (via drill 0.5)
  Top 0.406: OK202.14 73.34,8.24 72.07,9.51 68.58,9.51 66.99,11.09 v66.99,24.75 | v56.52,24.75 v56.52,37.13 | v37.15,37.13 v37.15,35.86
  Bottom 0.406: v66.99,24.75 v56.52,24.75 | v56.52,37.13 v37.15,37.13 | v37.15,35.86 IC101.17
I07  (via drill 0.5)
  Top 0.406: OK202.16 78.42,8.55 77.79,9.19 73.98,9.19 72.71,10.46 70.17,10.46 69.53,11.09 v69.53,25.7 | v57.47,25.7 v57.47,34.59 | v37.15,34.59 v37.15,33.32
  Bottom 0.406: v69.53,25.7 v57.47,25.7 | v57.47,34.59 v37.15,34.59 | v37.15,33.32 IC101.18
LED-G
  Bottom 0.406: R103.1 31.11,73.01 32.07,73.96 IC101.2
LED-R
  Bottom 0.406: R102.1 31.11,70.15 32.38,68.88 IC101.4
MISO  (via drill 0.5)
  Top 0.406: IC104.15 v39.69,18.71 39.69,19.03 40.96,20.3 v40.96,61.26 | SV101.1 v52.7,18.71 | IC103.2 44.77,13 46.04,14.27 46.04,18.08 v45.4,18.71
  Bottom 0.406: v40.96,61.26 IC101.7 | v52.7,18.71 v45.4,18.71 v39.69,18.71
MOSI  (via drill 0.5)
  Top 0.406: v38.42,63.8 38.42,20.3 37.15,19.03 IC104.14 37.15,9.51 v39.69,6.97 IC103.5
  Bottom 0.406: v38.42,63.8 IC101.6 | SV101.4 53.98,9.82 52.07,9.82 50.48,8.24 40.96,8.24 v39.69,6.97
N$1  (via drill 0.5)
  Top 0.61: IC104.1 v47.31,19.98 | v33.34,19.98 33.34,13.63 IC105.1
  Bottom 0.61: v47.31,19.98 v33.34,19.98
N$2  (via drill 0.5)
  Top 0.61: IC104.2 v44.77,21.25 | v28.26,21.25 28.26,13.63 IC105.4
  Bottom 0.61: v44.77,21.25 v28.26,21.25
N$3  (via drill 0.5)
  Top 0.813: X101.3 3.11,8.93 2.22,9.82 v2.22,53
  Bottom 0.813: v2.22,53 OK101.1 24.77,53 27.62,55.86 R109.1
N$5
  Top 0.813: OK101.3 28.57,48.88 R108.1
N$6
  Top 1.27: C105.1 30.48,80.62 V101.IN
  Bottom 1.27: D102.C 29.84,86.34 V101.IN | C105.1 42.55,80.62 C106.+
N$9
  Bottom 0.813: R102.2 12.38,70.15 7.94,74.59 D101.AR
N$13
  Bottom 0.813: R103.2 13.65,73.01 6.99,79.67 D101.AG
N$24  (via drill 0.5)
  Top 0.61: RN202.4 v70.8,33.95
  Bottom 0.61: v70.8,33.95 D207.C
  Bottom 1.27: D207.C 82.23,33.95 84.77,31.41 84.77,28.55 87.31,26.02 93.03,26.02 94.61,24.43 X204.1
N$25  (via drill 0.5)
  Top 0.61: RN202.2 75.88,16.81 74.61,15.54 v74.61,10.46 | v82.55,10.46 v82.55,19.03
  Bottom 0.61: v74.61,10.46 v82.55,10.46
  Bottom 1.27: D208.C 80.64,27.6 82.55,25.7 v82.55,19.03 82.55,18.39 84.77,16.17 87.95,16.17 92.71,11.41 X204.3
N$26  (via drill 0.5)
  Top 0.61: RN202.8 v60.64,20.93 | v73.34,20.93 v73.34,46.65
  Bottom 0.61: v60.64,20.93 v73.34,20.93 | v73.34,46.65 D205.C
  Bottom 1.27: D205.C 82.87,46.65 83.82,47.6 93.34,47.6 94.61,46.33 X203.1
N$27  (via drill 0.5)
  Top 0.61: RN202.6 v65.72,19.66 | v72.07,19.66 v72.07,40.3
  Bottom 0.61: v65.72,19.66 v72.07,19.66 | v72.07,40.3 D206.C
  Bottom 1.27: D206.C 86.04,40.3 92.39,33.95 X203.3
N$28  (via drill 0.5)
  Top 0.61: RN201.4 68.9,93.64 v68.9,59.35
  Bottom 0.61: v68.9,59.35 D203.C
  Bottom 1.27: D203.C 81.6,59.35 84.77,62.53 88.27,62.53 92.08,66.34 X202.1
N$29  (via drill 0.5)
  Top 0.61: RN201.2 73.98,93.64 73.98,88.56 74.93,87.61 81.28,87.61 82.87,86.02 v82.87,53
  Bottom 0.61: v82.87,53 D204.C
  Bottom 1.27: D204.C 84.77,53 85.41,52.37 93.03,52.37 94.61,53.95 X202.3
N$30  (via drill 0.5)
  Top 0.61: v71.44,72.05 v71.44,87.61 | v58.42,87.61 58.42,93.33 RN201.8
  Bottom 0.61: D201.C v71.44,72.05 | v71.44,87.61 v58.42,87.61
  Bottom 1.27: X201.1 93.98,88.88 90.49,85.39 85.41,85.39 83.5,83.48 83.5,73.96 81.92,72.37 79.69,72.37 D201.C
N$42
  Bottom 0.61: OK202.2 75.88,14.27 78.42,16.81 RN202.1
N$43
  Bottom 0.61: OK202.4 70.8,14.27 73.34,16.81 RN202.3
N$44
  Bottom 0.61: OK202.6 65.72,14.27 68.26,16.81 RN202.5
N$45
  Bottom 0.61: OK202.8 60.64,14.27 63.18,16.81 RN202.7
N$46
  Top 0.61: OK201.2 75.25,91.74 77.79,94.28 RN201.1
N$47  (via drill 0.5)
  Top 0.61: v67.63,65.7 67.63,73.96 66.36,75.23 66.36,86.66 63.82,89.2 63.82,93.64 RN201.6
  Bottom 0.61: D202.C v67.63,65.7
  Bottom 1.27: X201.3 93.66,78.72 91.12,76.18 91.12,75.23 81.92,66.02 79.69,66.02 D202.C
N$48
  Top 0.61: OK201.4 70.17,91.74 72.71,94.28 RN201.3
N$64
  Top 0.61: OK201.6 65.09,91.74 67.63,94.28 RN201.5
N$65
  Top 0.61: OK201.8 60.01,91.74 62.55,94.28 RN201.7
O00  (via drill 0.5)
  Top 0.406: v70.17,74.28 v70.17,48.56
  Bottom 0.406: LED201.K 83.19,87.61 81.92,86.34 81.92,75.55 80.64,74.28 v70.17,74.28 | v70.17,48.56 IC101.29
O01  (via drill 0.5)
  Top 0.406: v72.71,69.2 v72.71,62.53 | v59.69,62.53 v59.69,46.02
  Bottom 0.406: LED205.K 87.95,75.55 81.6,69.2 v72.71,69.2 | v72.71,62.53 v59.69,62.53 | v59.69,46.02 IC101.28
O02  (via drill 0.5)
  Top 0.406: v67.63,61.26 v67.63,43.48
  Bottom 0.406: LED202.K 84.45,65.07 80.64,61.26 v67.63,61.26 | v67.63,43.48 IC101.27
O03  (via drill 0.5)
  Top 0.406: v60.96,54.91 v60.96,40.94
  Bottom 0.406: LED206.K v60.96,54.91 | v60.96,40.94 IC101.26
O04
  Bottom 0.406: LED203.K 71.44,42.84 66.99,38.4 IC101.25
O05
  Bottom 0.406: LED207.K 86.36,32.68 82.55,36.49 60.33,36.49 59.69,35.86 IC101.24
O06  (via drill 0.5)
  Top 0.406: LED204.K 86.04,20.3 85.09,21.25 85.09,28.55 v82.23,31.41
  Bottom 0.406: v82.23,31.41 53.98,31.41 52.07,33.32 IC101.23
O07  (via drill 0.5)
  Top 0.406: LED208.K 84.77,10.14 83.82,11.09 83.82,27.6 v81.6,29.82
  Bottom 0.406: v81.6,29.82 51.75,29.82 50.8,30.78 IC101.22
PLUGGED  (via drill 0.5)
  Top 0.406: v13.02,71.73 13.02,83.1 CON101.3
  Bottom 0.406: IC101.39 39.37,73.96 38.1,75.23 27.94,75.23 24.13,71.42 13.34,71.42 v13.02,71.73
Q-CLK
  Bottom 0.61: IC101.13 33.34,46.02 30.8,43.48 30.8,31.41 28.89,29.51 QG101.8 28.89,26.65 29.53,26.02 IC104.8
SCK  (via drill 0.5)
  Top 0.406: IC104.13 v34.61,17.76 34.61,19.03 35.88,20.3 v35.88,58.72 | IC103.6 42.23,8.55 v43.5,9.82 v43.5,17.76
  Bottom 0.406: v35.88,58.72 IC101.8 | v43.5,17.76 v34.61,17.76 | SV101.3 51.44,11.09 50.16,9.82 v43.5,9.82
SPG
  Top 0.813: R107.1 R106.2
  Bottom 0.813: R106.2 53.02,81.9 49.21,78.09 49.21,76.81 IC101.40
V+  (via drill 0.5)
  Top 0.813: DC201.4 v56.2,42.21 | v59.05,42.21 v59.05,11.73
  Bottom 0.61: 63.82,11.73 63.18,11.73
  Bottom 0.813: OK202.1 78.42,11.73 73.34,11.73 | 73.34,11.73 68.26,11.73 | 68.26,11.73 63.82,11.73 v59.05,11.73 | 63.18,11.73 OK202.7 | OK202.3 73.34,11.73 | OK202.5 68.26,11.73 | OK201.1 77.79,89.2 72.71,89.2 | 72.71,89.2 67.63,89.2 | 67.63,89.2 62.55,89.2 | 62.55,89.2 OK201.7 | OK201.5 67.63,89.2 | OK201.3 72.71,89.2 | 62.55,89.2 55.24,89.2 54.61,88.56 54.61,78.72 51.12,75.23 51.12,70.78 51.75,70.15 C201.1 | v56.2,42.21 v59.05,42.21
  Bottom 1.27: C201.1 DC201.4
V-NETZTEIL1
  Bottom 1.27: CON101.1 19.37,90.47 22.23,93.33 D103.A

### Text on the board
Bottom: MBCAN-Projekt | (c) Dr.-Ing. Th. Wiesner | 06.01.2024 | mbc88ac.brd | bottom
tNames: HW: 24.01.06 | +18V | DC | Status | (c) Dr.-Ing. Th. Wiesner | MBCAN-Projekt | IN | OUT | mbc-88-AC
